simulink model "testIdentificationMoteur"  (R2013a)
settings: Solver=ode45  StartTime=0  StopTime=1  FixedStep=1e-3  MaxStep=SimParam.Te  RelTol=1e-8  AbsTol=1e-9
PreLoadFcn:
  | warning('off','sm:sli:setup:compile:LocalSolverNotSupported')
model workspace (MAT data in the model file):
  handle : class17 (value not decoded)
  handle : class17 (value not decoded)
undefined symbols (not defined in the file or in its folder): SimParam

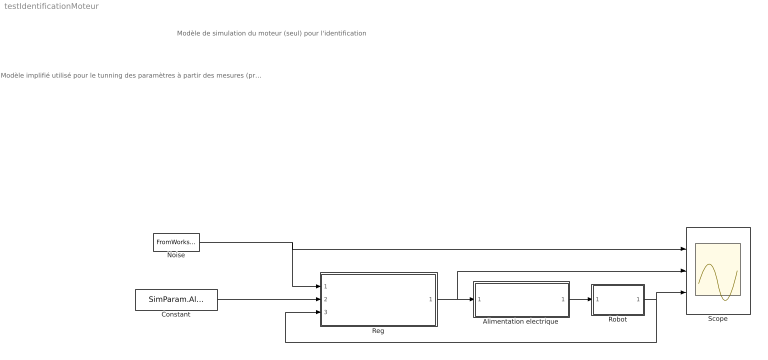
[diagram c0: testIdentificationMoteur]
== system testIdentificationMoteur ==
  note: Modèle de simulation du moteur (seul) pour l'identification
  note: Modèle implifié utilisé pour le tunning des paramètres à partir des mesures (prbs) effectuée sur le robot - Régulateur PID simple avec quantification codeur - Alimentation éléctrique modélisée par une fonction de transfert d'ordre deux avec delais (delais du contrôle) - Méchanique comprennant uniquement un modèle rigide du moteur (inertie + frottement) + frottement sec - Signaux d'exitation comprennant un bruit blanc et un signal cyclique (PRBS)
  Alimentation electrique : Subsystem
  Constant : Constant  Value=SimParam.Alpha_c
  Noise : FromWorkspace  VariableName=Noise  SampleTime=SimParam.Te  Interpolate=off  OutputAfterFinalValue=Holding final value
  Reg : Subsystem
  Robot : Subsystem
  Scope : Scope  NumInputPorts=3
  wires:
  Noise/1 -> Reg/1(Noise), Scope/1
  Alimentation electrique/1(Torque_out) -> Robot/1(In1)
  Robot/1(Out1) -> Scope/3, Reg/3(Alpha)
  Reg/1(Torque) -> Scope/2, Alimentation electrique/1(Torque_in)
  Constant/1 -> Reg/2(Alpha_c)

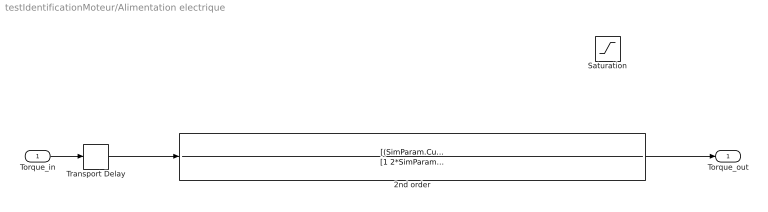
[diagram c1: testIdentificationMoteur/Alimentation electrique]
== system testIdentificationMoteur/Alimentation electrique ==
  Torque_in : Inport
  2nd order : TransferFcn  Numerator=[(SimParam.CurrentLoop.f0*2*pi)^2]  Denominator=[1 2*SimParam.CurrentLoop.Cr*(SimParam.CurrentLoop.f0*2*pi) (SimParam.CurrentLoop.f0*2*pi)^2]
  Saturation : Saturate  Commented=on  UpperLimit=20  LowerLimit=-20
  Transport Delay : TransportDelay  DelayTime=SimParam.tau
  Torque_out : Outport
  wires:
  Torque_in/1 -> Transport Delay/1
  Transport Delay/1 -> 2nd order/1
  2nd order/1 -> Torque_out/1

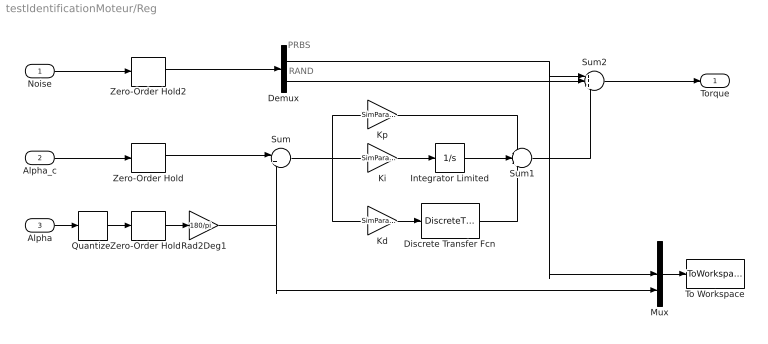
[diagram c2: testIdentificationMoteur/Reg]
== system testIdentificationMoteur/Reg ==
  note: RAND
  note: PRBS
  Noise : Inport
  Alpha_c : Inport  Port=2
  Alpha : Inport  Port=3
  Demux : Demux  Outputs=2
  Discrete Transfer Fcn : DiscreteTransferFcn  Numerator=[1 0 -1]  Denominator=[2 0 0]
  Integrator Limited : Integrator  LimitOutput=on  UpperSaturationLimit=1  LowerSaturationLimit=-1
  Kd : Gain  Gain=SimParam.Control.Kd/SimParam.Te
  Ki : Gain  Gain=SimParam.Control.Ki*SimParam.Te
  Kp : Gain  Gain=SimParam.Control.Kp
  Mux : Mux  Inputs=3
  Quantizer : Quantizer  QuantizationInterval=SimParam.CoderResol
  Rad2Deg1 : Gain  Gain=180/pi
  Sum : Sum  Inputs=|+-
  Sum1 : Sum  Inputs=+++
  Sum2 : Sum  Inputs=+++
  To Workspace : ToWorkspace  VariableName=simout  SampleTime=SimParam.Te  SaveFormat=Structure With Time
  Zero-Order Hold : ZeroOrderHold  SampleTime=SimParam.Te
  Zero-Order Hold1 : ZeroOrderHold  SampleTime=SimParam.Te
  Zero-Order Hold2 : ZeroOrderHold  SampleTime=SimParam.Te
  Torque : Outport
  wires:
  Alpha_c/1 -> Zero-Order Hold/1
  Kd/1 -> Discrete Transfer Fcn/1
  Mux/1 -> To Workspace/1
  Zero-Order Hold/1 -> Sum/1
  Alpha/1 -> Quantizer/1
  Quantizer/1 -> Zero-Order Hold1/1
  Noise/1 -> Zero-Order Hold2/1
  Discrete Transfer Fcn/1 -> Sum1/3
  Kp/1 -> Sum1/1
  Sum1/1 -> Sum2/3
  Demux/1 -> Mux/2, Sum2/1
  Sum2/1 -> Torque/1
  Ki/1 -> Integrator Limited/1
  Integrator Limited/1 -> Sum1/2
  Sum/1 -> Ki/1, Kp/1, Kd/1
  Zero-Order Hold1/1 -> Rad2Deg1/1
  Rad2Deg1/1 -> Mux/3, Sum/2
  Demux/2 -> Sum2/2
  Zero-Order Hold2/1 -> Demux/1

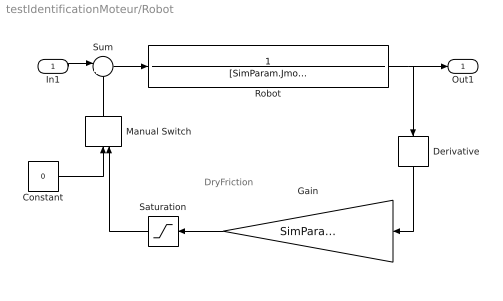
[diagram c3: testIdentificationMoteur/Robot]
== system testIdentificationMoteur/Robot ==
  note: DryFriction
  In1 : Inport
  Constant : Constant  Value=0
  Derivative : Derivative
  Gain : Gain  Gain=SimParam.CdmotorSlope
  Manual Switch : ManualSwitch  CurrentSetting=0
  Robot : TransferFcn  Numerator=1  Denominator=[SimParam.Jmotor SimParam.Cmotor 0]
  Saturation : Saturate  UpperLimit=SimParam.Cdmotor  LowerLimit=-SimParam.Cdmotor
  Sum : Sum  Inputs=|+-
  Out1 : Outport
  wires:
  Robot/1 -> Derivative/1, Out1/1
  In1/1 -> Sum/1
  Sum/1 -> Robot/1
  Derivative/1 -> Gain/1
  Gain/1 -> Saturation/1
  Saturation/1 -> Manual Switch/2
  Constant/1 -> Manual Switch/1
  Manual Switch/1 -> Sum/2
